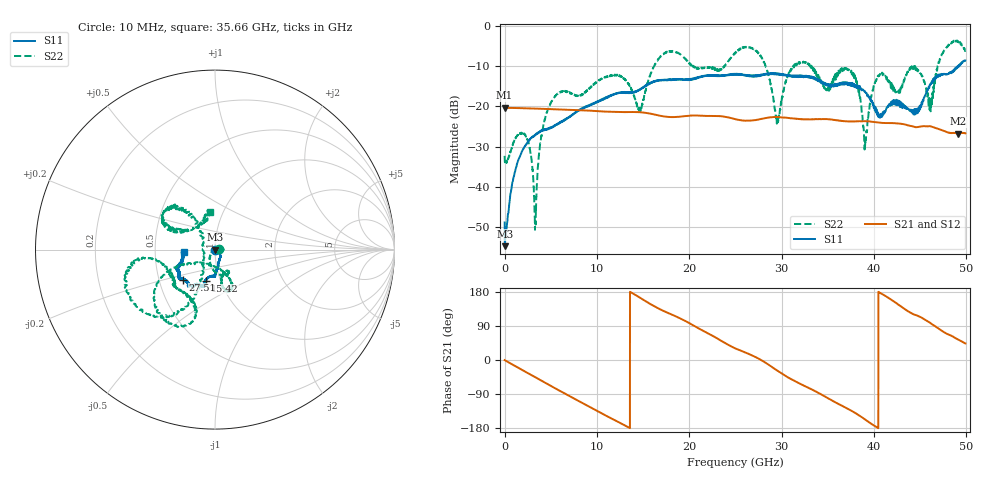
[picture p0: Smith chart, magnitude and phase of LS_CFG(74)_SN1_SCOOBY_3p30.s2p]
!Keysight Technologies,N5245B,MY58422026,A.13.80.08
!Date: Thursday, March 19, 2020 23:50:13
!Correction: S11(Full 2 Port(1,2))
!S21(Full 2 Port(1,2))
!S12(Full 2 Port(1,2))
!S22(Full 2 Port(1,2))
!S2P File: Measurements: S11, S21, S12, S22:
# Hz S DB R 50.0
!freq dBS11 angS11 dBS21 angS21 dBS12 angS12 dBS22 angS22
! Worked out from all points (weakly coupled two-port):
!   4991 points, 10 MHz to 49.91 GHz, reference 50 ohm
!   highest |S21| = -20.34 dB at 10 MHz (marker M1); lowest = -26.8 dB at 49.11 GHz (marker M2)
!   lowest |S11| = -54.7 dB at 40 MHz (marker M3), VSWR 1.00, Z = 50.2 + j0.00653 ohm
!   |S11| at or under -10 dB: start of sweep to 49.12 GHz; 49.16785 GHz to 49.22354 GHz (55.69 MHz wide, 0.113 % of centre)
!   |S22| runs from -50.6 to -3.7 dB; largest |S21 - S12| = 0.00096
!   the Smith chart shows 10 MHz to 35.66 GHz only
!   S11 on the Smith chart (normalised r, x): 10 MHz: 1.00, -0.01; 15.42 GHz: 0.85, -0.31; 27.51 GHz: 0.67, -0.24; 35.66 GHz: 0.70, -0.01
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1e7  -48.81 -52.0  -20.34 -0.3  -20.33 -0.3  -32.29 1.9
4e7  -54.70 2.0  -20.35 -0.7  -20.34 -0.6  -33.87 -4.9
2.21e9  -29.84 -40.8  -20.49 -30.4  -20.48 -30.3  -27.00 8.1
3.33e9  -27.00 -48.3  -20.56 -45.4  -20.56 -45.4  -48.87 126.1
4.87e9  -25.36 -58.8  -20.69 -66.4  -20.69 -66.4  -19.87 -100.5
8.33e9  -20.75 -79.7  -20.97 -112.4  -20.97 -112.3  -17.16 -68.7
1.542e10  -14.81 -106.7  -21.66 153.2  -21.66 153.3  -14.95 -154.2
1.665e10  -13.63 -106.9  -22.24 136.2  -22.23 136.3  -8.31 -148.0
2.496e10  -12.10 -127.0  -23.14 31.1  -23.13 31.3  -6.85 -170.4
2.751e10  -12.25 -136.5  -23.26 3.6  -23.27 3.9  -6.73 -125.3
2.956e10  -11.88 -142.7  -22.67 -28.4  -22.66 -28.1  -23.12 -179.5
3.104e10  -12.44 -147.0  -22.96 -50.6  -22.97 -50.3  -10.74 129.4
3.328e10  -12.80 -156.9  -23.21 -78.0  -23.21 -77.5  -10.40 155.9
3.566e10  -15.05 -176.8  -23.33 -109.4  -23.28 -108.9  -13.19 97.3
3.78e10  -14.95 177.5  -23.76 -137.2  -23.70 -137.3  -11.86 134.3
3.904e10  -16.29 173.7  -23.67 -156.8  -23.65 -157.0  -30.13 -129.2
4.021e10  -21.36 162.4  -23.94 -175.9  -23.92 -176.1  -13.62 -5.9
4.16e10  -19.63 105.0  -24.16 163.6  -24.18 163.6  -13.89 24.8
4.445e10  -21.20 50.7  -25.15 119.3  -25.16 119.6  -10.22 -16.1
4.614e10  -14.48 5.7  -24.95 97.2  -24.96 97.4  -20.85 -47.6
4.911e10  -10.14 -14.5  -26.76 54.0  -26.77 54.1  -3.84 -44.5
4.991e10  -8.61 -14.6  -26.67 43.7  -26.69 43.8  -6.21 -29.2
